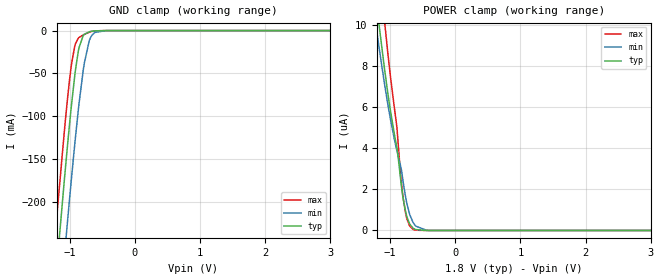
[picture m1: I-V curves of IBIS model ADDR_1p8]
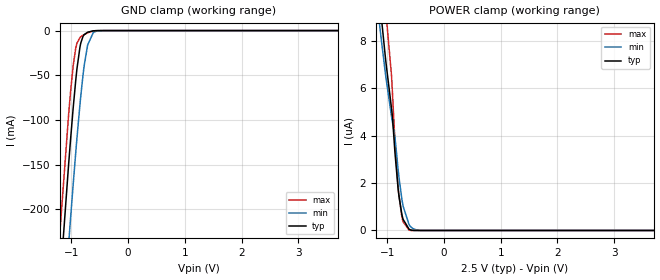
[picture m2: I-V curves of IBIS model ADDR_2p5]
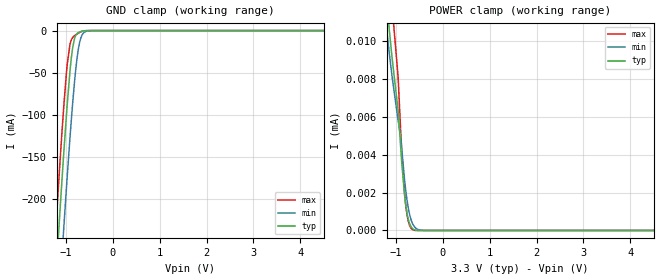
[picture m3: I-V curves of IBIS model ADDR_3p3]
| Texas Instruments Incorporated
| Low Power Humidity and Temperature Digital Sensors
| Marketing part#   Voltage Range   Package-type   #pins/pkg drawing
| HDC2010YPA   1.62V - 3.6V   BGA   6-pin YPA
[IBIS Ver]   4.1
[File name]   hdc2010.ibs
[File Rev]   1.0
[Date]   01/18/2017
[Source]   Model built from spectre simulations at:
   Texas Instruments Incorporated.
   Webench Design Center
   12500 TI Blvd
   Dallas, TX -75243
   For Support e-mail: elab_ibis@list.ti.com
[Notes]   Revision History
   Rev 1.0: 01/18/2017
   - Non monotonic behavior result of circuit behavior
   - ccomp values are based on PVT settings:
   MIN: Low Voltage, High Temperature, Weak Process
   TYP: Nominal Voltage, Nominal Temperature, Nominal Process
   MAX: High Voltage, Low Temperature, Fast Process
   - C_comp although listed in numerical order of value are obtained from varying PVT conditions.
   For PVT conditions for each specific value, refer to the buffer description under respective [Model].
   IBIS model user is responsible for using appropriate C_comp to simulate for Signal Integrity.
[Disclaimer]  This model is designed as an aid for customers of Texas Instruments
 TI and its licensors and suppliers make no warranties, either expressed
 or implied, with respect to this  model, including the warranties of
 merchantability or fitness for a particular purpose.
 The model is provided solely on an "as is" basis. The entire risk as to
 its quality and performance is with the customer.
[Copyright] (C)Copyright 2017 Texas Instruments Incorporated.
   All rights reserved.
[Component]   HDC2010YPA
[Manufacturer]  Texas Instruments Incorporated
[Package]   |6-pin BGA YPA package
|   typ   min   max
R_pkg   0.005   0.005   0.005
L_pkg   0.20nH   0.2nH   0.2nH
C_pkg   0.6pF   0.6pF   0.6pF
[Pin]   signal_name   model_name   R_pin   L_pin   C_pin
A1   VDD   POWER   0.005   0.2nH   0.6pF
A2   SDA   SDA   0.005   0.2nH   0.6pF
B1   ADDR   ADDR   0.005   0.2nH   0.6pF
B2   SCL   SCL   0.005   0.2nH   0.6pF
C1   GND   GND   0.005   0.2nH   0.6pF
C2   DRDY/INT   DRDY   0.005   0.2nH   0.6pF
[Model Selector] SDA
SDA_3p3   3.3V OPEN DRAIN I/O
SDA_2p5   2.5V OPEN DRAIN I/O
SDA_1p8   1.8V OPEN DRAIN I/O
[Model Selector] DRDY
DRDY_3p3   3.3V I/O
DRDY_2p5   2.5V I/O
DRDY_1p8   1.8V I/O
[Model Selector] SCL
SCL_3p3   3.3V INPUT
SCL_2p5   2.5V INPUT
SCL_1p8   1.8V INPUT
[Model Selector] ADDR
ADDR_3p3   3.3V INPUT
ADDR_2p5   2.5V INPUT
ADDR_1p8   1.8V INPUT
| Models and submodels in the file (12): ADDR_1p8 (Input), ADDR_2p5 (Input), ADDR_3p3 (Input), DRDY_1p8 (I/O), DRDY_2p5 (I/O), DRDY_3p3 (I/O), SCL_1p8 (Input), SCL_2p5 (Input), SCL_3p3 (Input), SDA_3p3 (I/O_open_drain), SDA_2p5 (I/O_open_drain), SDA_1p8 (I/O_open_drain)
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|   Model IN_3P3V
[Model]   ADDR_1p8
Model_type   Input
Vinl = 0.54
Vinh = 1.26
|   typ   min   max
|   (nom PVT)   (slow PVT)   (fast PVT)
C_comp   0.684p   0.665p   0.698p
[Model spec]
|subparameter
Vinl   0.54   0.486   0.594
Vinh   1.26   1.134   1.386
[Voltage Range]   1.8   1.62   1.98
[Temperature Range]   27   125   -40
[Power Clamp Reference]   1.8   1.62   1.98
[GND Clamp Reference]   0   0   0
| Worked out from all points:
|   GND clamp passes 1 mA (typ) near -0.68 V on its own axis
[GND Clamp]
|   Voltage   I(typ)   I(min)   I(max)
-1.8V     -845.7mA   -933.3mA   -789.9mA
-1.222V   -299.8mA   -390.8mA   -241.2mA
-1.184V   -265.8mA   -356.7mA   -207.2mA
-1.076V   -171.4mA   -261.4mA   -114.6mA
-1.033V   -135.6mA   -224.4mA   -80.86mA
-973.8mV  -89.32mA   -175.1mA   -41.3mA
-919.8mV  -52.43mA   -132.5mA   -18.12mA
-855mV    -20.03mA   -85.72mA   -8.039mA
-790.2mV  -5.799mA   -46.45mA   -5.026mA
-660.6mV  -782uA     -5.921mA   -1.008mA
-444.6mV  -4.712uA   -64.2uA    -1.272uA
3.6V      0A         0A         0A
[POWER Clamp]
|   Voltage   I(typ)   I(min)   I(max)
-1.8V     30.32uA    25.8uA     39.25uA
-1.201V   10.83uA    9.593uA    14.1uA
-1.174V   10.1uA     8.984uA    13.14uA
-1.082V   7.756uA    7.039uA    10.05uA
-995.4mV  5.828uA    5.418uA    7.494uA
-898.2mV  4.06uA     3.903uA    5.074uA
-849.6mV  2.774uA    3.274uA    3.086uA
-801mV    1.567uA    2.37uA     1.583uA
-741.6mV  653.5nA    1.287uA    547.5nA
-649.8mV  117.3nA    399.5nA    58.47nA
-379.8mV  0A         469.3pA    0A
3.6V      0A         0A         0A
[Model]   ADDR_2p5
Model_type   Input
Vinl = 0.75
Vinh = 1.75
|   typ   min   max
|   (nom PVT)   (slow PVT)   (fast PVT)
C_comp   0.671p   0.651p   0.685p
[Model spec]
|subparameter
Vinl   0.75   0.675   0.825
Vinh   1.75   1.575   1.925
[Voltage Range]   2.5   2.25   2.75
[Temperature Range]   27   125   -40
[Power Clamp Reference]   2.5   2.25   2.75
[GND Clamp Reference]   0   0   0
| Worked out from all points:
|   GND clamp passes 1 mA (typ) near -0.66 V on its own axis
[GND Clamp]
|   Voltage   I(typ)   I(min)   I(max)
-2.5V     -1.528A    -1.611A    -1.475A
-1.218V   -295.6mA   -386.5mA   -237mA
-1.052V   -151.4mA   -240.8mA   -95.57mA
-1.038V   -139.1mA   -228mA     -84.08mA
-970mV    -86.53mA   -172mA     -39.19mA
-925mV    -55.68mA   -136.5mA   -19.67mA
-850mV    -18.28mA   -82.37mA   -7.69mA
-775mV    -4.465mA   -38.81mA   -4.517mA
-715mV    -1.831mA   -16.17mA   -2.451mA
-617.5mV  -351.5uA   -2.471mA   -388.5uA
-475mV    -11.29uA   -123.7uA   -4.166uA
5V        0A         0A         0A
[POWER Clamp]
|   Voltage   I(typ)   I(min)   I(max)
-2.5V     57.7uA     48.77uA    74.14uA
-1.135V   9.708uA    8.634uA    12.66uA
-1.113V   9.138uA    8.16uA     11.91uA
-1.022V   7.033uA    6.4uA      9.118uA
-925mV    5.118uA    4.783uA    6.483uA
-910mV    4.785uA    4.564uA    5.781uA
-865mV    3.248uA    3.915uA    3.704uA
-797.5mV  1.495uA    2.291uA    1.506uA
-722.5mV  471.7nA    1.026uA    367.4nA
-617.5mV  54.78nA    247.9nA    17.46nA
-400mV    0A         417.4pA    0A
5V        0A         0A         0A
[Model]   ADDR_3p3
Model_type   Input
Vinl = 0.99
Vinh = 2.31
|   typ   min   max
|   (nom PVT)   (slow PVT)   (fast PVT)
C_comp   0.655p   0.636p   0.670p
[Model spec]
|subparameter
Vinl   0.99   0.90   1.08
Vinh   2.31   2.10   2.52
[Voltage Range]   3.3   3   3.6
[Temperature Range]   27   125   -40
[Power Clamp Reference]   3.3   3   3.6
[GND Clamp Reference]   0   0   0
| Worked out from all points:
|   GND clamp passes 1 mA (typ) near -0.68 V on its own axis
[GND Clamp]
|   Voltage   I(typ)   I(min)   I(max)
-3.3V     -2.315A    -2.395A    -2.265A
-1.221V   -298.7mA   -389.7mA   -240.1mA
-1.122V   -210.6mA   -301.2mA   -152.7mA
-1.053V   -151.6mA   -241mA     -95.73mA
-973.5mV  -89.1mA    -174.9mA   -41.13mA
-884.4mV  -32.65mA   -106.2mA   -10.97mA
-815.1mV  -9.292mA   -60.38mA   -5.915mA
-755.7mV  -3.3mA     -30.16mA   -3.853mA
-706.2mV  -1.61mA    -13.9mA    -2.172mA
-627mV    -423.7uA   -3.005mA   -488.4uA
-468.6mV  -9.421uA   -107.8uA   -3.257uA
6.6V      0A         0A         0A
[POWER Clamp]
|   Voltage   I(typ)   I(min)   I(max)
-3.3V     91.61uA    77.46uA    117.1uA
-1.28V    14.43uA    12.54uA    18.85uA
-1.142V   10.6uA     9.362uA    13.83uA
-1.082V   9.119uA    8.131uA    11.88uA
-953.7mV  6.34uA     5.811uA    8.108uA
-894.3mV  4.253uA    4.853uA    5.028uA
-874.5mV  3.556uA    4.302uA    4.12uA
-795.3mV  1.449uA    2.229uA    1.462uA
-726mV    498.7nA    1.059uA    398.5nA
-627mV    66.24nA    280nA      23.45nA
-399.3mV  0A         0A         0A
6.6V      0A         0A         0A
